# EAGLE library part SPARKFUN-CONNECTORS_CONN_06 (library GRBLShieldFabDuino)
Multi connection point. Often used as Generic Header-pin footprint for 0.1 inch spaced/style header connections On any of the 0.1 inch spaced packages, you can populate with these: Break Away Headers - Straight (PRT-00116) Break Away Male Headers - Right Angle (PRT-00553) Female Headers (PRT-00115) Break Away Headers - Machine Pin (PRT-00117) Break Away Female Headers - Swiss Machine Pin (PRT-00743) Arduino Stackable Header - 6 Pin (PRT-09280) For SCREWTERMINALS and SPRING TERMINALS visit here: Screw Terimnals on SparkFun.com (5mm/3.5mm/2.54mm spacing) This device is also useful as a general connection point to wire up your design to another part of your project. Our various solder wires solder well into these plated through hole pads. Hook-Up Wire - Assortment (Stranded, 22 AWG) (PRT-11375) Hook-Up Wire - Assortment (Solid Core, 22 AWG) (PRT-11367) View the entire wire category on our website here
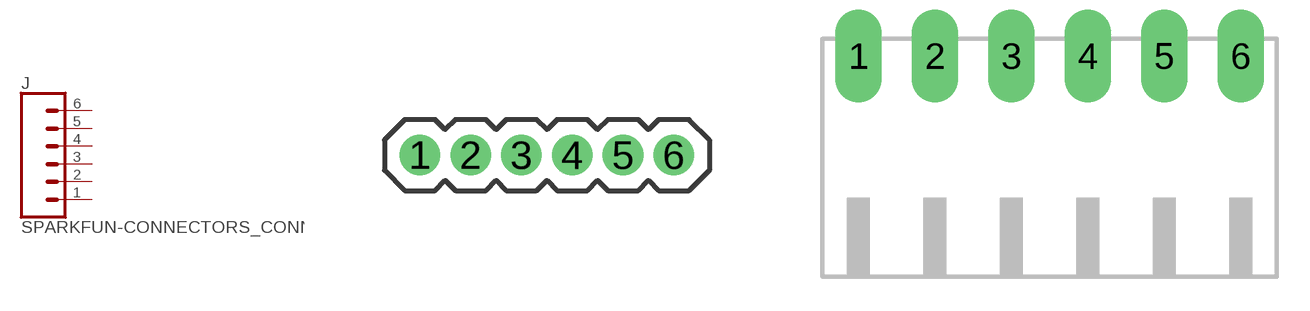
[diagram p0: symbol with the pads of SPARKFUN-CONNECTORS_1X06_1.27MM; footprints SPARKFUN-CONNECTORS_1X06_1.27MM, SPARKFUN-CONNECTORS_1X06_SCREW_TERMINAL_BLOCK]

Designator prefix J

## SPARKFUN-CONNECTORS_CONN_061.27MM  [SPARKFUN-CONNECTORS_1X06_1.27MM]
1  1  pas
2  2  pas
3  3  pas
4  4  pas
5  5  pas
6  6  pas

## SPARKFUN-CONNECTORS_CONN_062.5MM-6-90  [SPARKFUN-CONNECTORS_1X06_SCREW_TERMINAL_BLOCK]
Pads as for SPARKFUN-CONNECTORS_1X06_1.27MM

## SPARKFUN-CONNECTORS_CONN_063.5MM-6  [SPARKFUN-CONNECTORS_SCREWTERMINAL-3.5MM-6]
Pads as for SPARKFUN-CONNECTORS_1X06_1.27MM

## SPARKFUN-CONNECTORS_CONN_06FEMALE_LOCK  [SPARKFUN-CONNECTORS_1X06_FEMALE_LOCK.010]
Pads as for SPARKFUN-CONNECTORS_1X06_1.27MM

## SPARKFUN-CONNECTORS_CONN_06LOCK  [SPARKFUN-CONNECTORS_1X06_LOCK]
Pads as for SPARKFUN-CONNECTORS_1X06_1.27MM

## SPARKFUN-CONNECTORS_CONN_06LOCK_LONGPADS  [SPARKFUN-CONNECTORS_1X06_LOCK_LONGPADS]
Pads as for SPARKFUN-CONNECTORS_1X06_1.27MM

## SPARKFUN-CONNECTORS_CONN_06LONGPADS  [SPARKFUN-CONNECTORS_1X06_LONGPADS]
Pads as for SPARKFUN-CONNECTORS_1X06_1.27MM

## SPARKFUN-CONNECTORS_CONN_06NO_SILK_FEMALE_PTH (PROD_ID: CONN-08437)  [SPARKFUN-CONNECTORS_1X06_NO_SILK]
Pads as for SPARKFUN-CONNECTORS_1X06_1.27MM

## SPARKFUN-CONNECTORS_CONN_06NO_SILK_NO_POP  [SPARKFUN-CONNECTORS_1X06_NO_SILK]
Pads as for SPARKFUN-CONNECTORS_1X06_1.27MM

## SPARKFUN-CONNECTORS_CONN_06POGOPIN_HOLES_ONLY (PROD_ID: CONN-08437)  [SPARKFUN-CONNECTORS_1X06_HOLES_ONLY]
Pads as for SPARKFUN-CONNECTORS_1X06_1.27MM

## SPARKFUN-CONNECTORS_CONN_06POLAR  [SPARKFUN-CONNECTORS_MOLEX-1X6]
Pads as for SPARKFUN-CONNECTORS_1X06_1.27MM

## SPARKFUN-CONNECTORS_CONN_06POLAR_LOCK  [SPARKFUN-CONNECTORS_MOLEX-1X6_LOCK]
Pads as for SPARKFUN-CONNECTORS_1X06_1.27MM

## SPARKFUN-CONNECTORS_CONN_06RA  [SPARKFUN-CONNECTORS_MOLEX-1X6-RA]
Pads as for SPARKFUN-CONNECTORS_1X06_1.27MM

## SPARKFUN-CONNECTORS_CONN_06RA_LOCK  [SPARKFUN-CONNECTORS_MOLEX_1X6_RA_LOCK]
Pads as for SPARKFUN-CONNECTORS_1X06_1.27MM

## SPARKFUN-CONNECTORS_CONN_06SILK_FEMALE_PTH (PROD_ID: CONN-08437)  [SPARKFUN-CONNECTORS_1X06]
Pads as for SPARKFUN-CONNECTORS_1X06_1.27MM

## SPARKFUN-CONNECTORS_CONN_06SMD (PROD_ID: CONN-08971; VALUE: RA 6Pin SMD)  [SPARKFUN-CONNECTORS_1X06-SMD_RA_MALE]
Pads as for SPARKFUN-CONNECTORS_1X06_1.27MM

## SPARKFUN-CONNECTORS_CONN_06SMD-1MM (PROD_ID: CONN-08249; SF_ID: GPS-00579)  [SPARKFUN-CONNECTORS_1X06-1MM]
Pads as for SPARKFUN-CONNECTORS_1X06_1.27MM

## SPARKFUN-CONNECTORS_CONN_06SMD-FEMALE-V2 (PROD_ID: CONN-09668)  [SPARKFUN-CONNECTORS_1X06-SMD-FEMALE]
Pads as for SPARKFUN-CONNECTORS_1X06_1.27MM

## SPARKFUN-CONNECTORS_CONN_06SMD-STRAIGHT-ALT-FEMALE (PROD_ID: CONN-10203)  [SPARKFUN-CONNECTORS_1X06_SMD_STRAIGHT_ALT]
Pads as for SPARKFUN-CONNECTORS_1X06_1.27MM

## SPARKFUN-CONNECTORS_CONN_06SMD-STRAIGHT-COMBO-FEMALE (PROD_ID: CONN-10203)  [SPARKFUN-CONNECTORS_1X06_SMD_STRAIGHT_COMBO]
Pads as for SPARKFUN-CONNECTORS_1X06_1.27MM

## SPARKFUN-CONNECTORS_CONN_06SMD-STRAIGHT-FEMALE (PROD_ID: CONN-10203)  [SPARKFUN-CONNECTORS_1X06_SMD_STRAIGHT]
Pads as for SPARKFUN-CONNECTORS_1X06_1.27MM

## SPARKFUN-CONNECTORS_CONN_06SMD_MALE (PROD_ID: CONN-11293)  [SPARKFUN-CONNECTORS_1X06_SMD_MALE]
Pads as for SPARKFUN-CONNECTORS_1X06_1.27MM

## Footprint SPARKFUN-CONNECTORS_1X06_1.27MM (pad centres in mm)
Plated Through Hole - 6 Pin Specifications: Pin count:6 Pin pitch:1.27mm Example device(s): CONN_06
drill 0.508 pad 1: 1 0,0; 2 1.27,0; 3 2.54,0; 4 3.81,0; 5 5.08,0; 6 6.35,0

## Footprint SPARKFUN-CONNECTORS_1X06_SCREW_TERMINAL_BLOCK (pad centres in mm)
drill 1.422 long: 1 -8.75,5.25; 2 -5.25,5.25; 3 -1.75,5.25; 4 1.75,5.25; 5 5.25,5.25; 6 8.75,5.25

## Footprint SPARKFUN-CONNECTORS_SCREWTERMINAL-3.5MM-6 (pad centres in mm)
Screw Terminal 3.5mm Pitch -6 Pin PTH Specifications: Pin count: 6 Pin pitch: 3.5mm/138mil Datasheet referenced for footprint Example device(s): CONN_06
drill 1.2 pad 2.032 square: 1 0,0
drill 1.2 pad 2.032: 2 3.5,0; 3 7,0; 4 10.5,0; 5 14,0; 6 17.5,0

## Footprint SPARKFUN-CONNECTORS_1X06_FEMALE_LOCK.010 (pad centres in mm)
Plated Through Hole - 6 Pin Locking Header Includes silk outline for 6 pin female header Specifications: Pin count:6 Pin pitch:0.1" Datasheet referenced for footprint: Example device(s): CONN_06
drill 1.016 pad 1.88: 1 0,0.254; 2 2.54,-0.254; 3 5.08,0.254; 4 7.62,-0.254; 5 10.16,0.254; 6 12.7,-0.254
